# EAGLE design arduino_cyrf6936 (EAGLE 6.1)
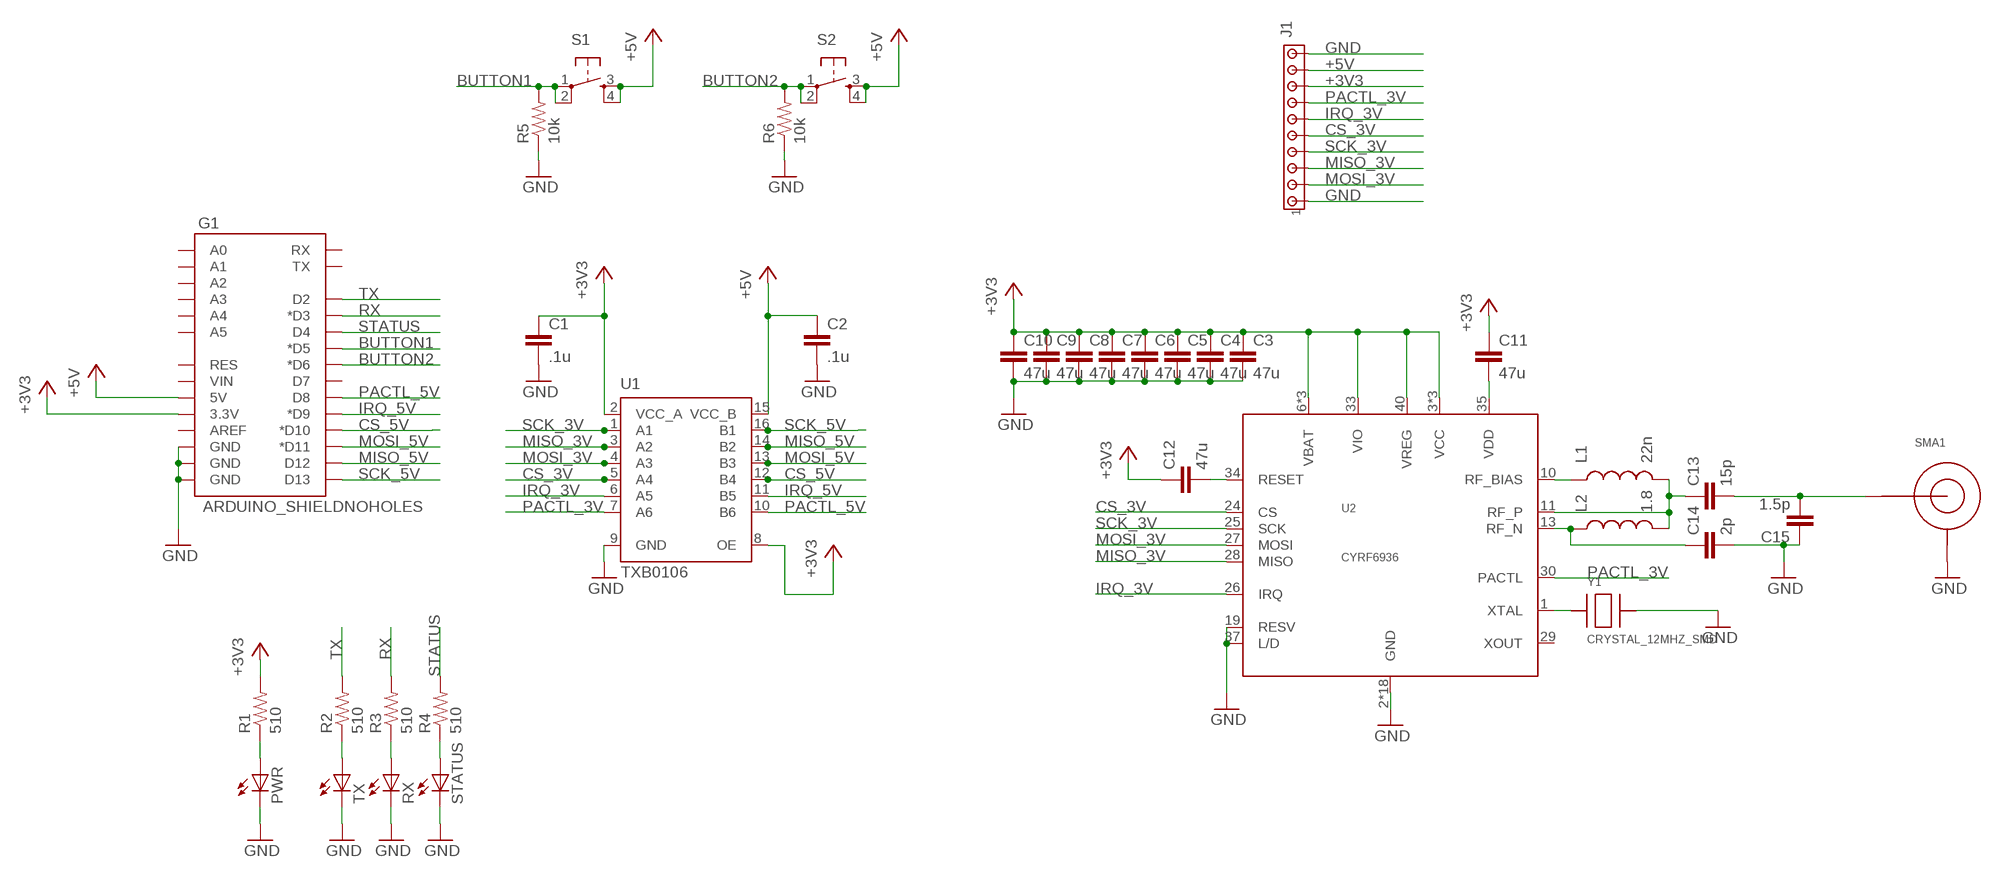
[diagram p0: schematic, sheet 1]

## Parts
C1  .1u  CAP0603-CAP  [0603-CAP]
C2  .1u  CAP0603-CAP  [0603-CAP]
C3  47u  CAP0603-CAP  [0603-CAP]
C4  47u  CAP0603-CAP  [0603-CAP]
C5  47u  CAP0603-CAP  [0603-CAP]
C6  47u  CAP0603-CAP  [0603-CAP]
C7  47u  CAP0603-CAP  [0603-CAP]
C8  47u  CAP0603-CAP  [0603-CAP]
C9  47u  CAP0603-CAP  [0603-CAP]
C10  47u  CAP0603-CAP  [0603-CAP]
C11  47u  CAP0603-CAP  [0603-CAP]
C12  47u  CAP0603-CAP  [0603-CAP]
C13  15p  CAP0402-CAP  [0402-CAP]
C14  2p  CAP0402-CAP  [0402-CAP]
C15  1.5p  CAP0402-CAP  [0402-CAP]
G1  ARDUINO_SHIELDNOHOLES  [DUEMILANOVE_SHIELD_NOHOLES]
J1  MTA10-100  [10X10MTA]
L1  22n  INDUCTOR0603  [0603]
L2  1.8  INDUCTOR0402  [C0402]
PWR  LED0603  [LED-0603]
R1  510  RESISTOR0603-RES  [0603-RES]
R2  510  RESISTOR0603-RES  [0603-RES]
R3  510  RESISTOR0603-RES  [0603-RES]
R4  510  RESISTOR0603-RES  [0603-RES]
R5  10k  RESISTOR0603-RES  [0603-RES]
R6  10k  RESISTOR0603-RES  [0603-RES]
RX  LED0603  [LED-0603]
S1  TAC_SWITCHSMD  [TACTILE_SWITCH_SMD]
S2  TAC_SWITCHSMD  [TACTILE_SWITCH_SMD]
SMA1  SMA_EDGE  [SMA_EDGE]
STATUS  LED0603  [LED-0603]
TX  LED0603  [LED-0603]
U1  TXB0106  [TSSOP16]
U2  CYRF6936  [QFN40-6X6]
Y1  CRYSTAL_12MHZ_SMD  [SMD-4_5X3.2MM]

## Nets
+3V3: C1.1 C3.1 C4.1 C5.1 C6.1 C7.1 C8.1 C9.1 C10.1 C11.1 C12.1 G1.3.3V J1.8 R1.2 U1.2(VCC_A) U1.8(OE) U2.3(VCC) U2.6(VBAT) U2.7(VCC) U2.8(VBAT) U2.16(VCC) U2.33(VIO) U2.38(VBAT) U2.40(VREG)
+5V: C2.1 G1.5V J1.9 S1.3 S1.4 S2.3 S2.4 U1.15(VCC_B)
BUTTON1: G1.D5(*D5) R5.2 S1.1 S1.2
BUTTON2: G1.D6(*D6) R6.2 S2.1 S2.2
CS_3V: J1.5 U1.5(A4) U2.24(CS)
CS_5V: G1.D10(*D10) U1.12(B4)
GND: C1.2 C2.2 C3.2 C4.2 C5.2 C6.2 C7.2 C8.2 C9.2 C10.2 C14.2 C15.1 G1.GND@0(GND) G1.GND@1(GND) G1.GND@2(GND) J1.1 J1.10 PWR.C R5.1 R6.1 RX.C SMA1.GND1(SHIELD) SMA1.GND2(SHIELD) STATUS.C TX.C U1.9(GND) U2.2(GND) U2.4(GND) U2.5(GND) U2.9(GND) U2.12(GND) U2.14(GND) U2.15(GND) U2.17(GND) U2.18(GND) U2.19(RESV) U2.20(GND) U2.21(GND) U2.22(GND) U2.23(GND) U2.31(GND) U2.32(GND) U2.36(GND) U2.37(L/D) U2.39(GND) U2.EXP(GND) Y1.P$3
IRQ_3V: J1.6 U1.6(A5) U2.26(IRQ)
IRQ_5V: G1.D9(*D9) U1.11(B5)
MISO_3V: J1.3 U1.3(A2) U2.28(MISO)
MISO_5V: G1.D12 U1.14(B2)
MOSI_3V: J1.2 U1.4(A3) U2.27(MOSI)
MOSI_5V: G1.D11(*D11) U1.13(B3)
N$1: PWR.A R1.1
N$2: R2.1 TX.A
N$3: R3.1 RX.A
N$4: R4.1 STATUS.A
N$5: L1.1 U2.10(RF_BIAS)
N$6: C13.1 L1.2 L2.2 U2.11(RF_P)
N$7: C11.2 U2.35(VDD)
N$8: C12.2 U2.34(RESET)
N$9: C14.1 L2.1 U2.13(RF_N)
N$10: U2.1(XTAL) Y1.P$1
N$11: C13.2 C15.2 SMA1.SIGNAL(CENTER)
PACTL_3V: J1.7 U1.7(A6) U2.30(PACTL)
PACTL_5V: G1.D8 U1.10(B6)
RX: G1.D3(*D3) R3.2
SCK_3V: J1.4 U1.1(A1) U2.25(SCK)
SCK_5V: G1.D13 U1.16(B1)
STATUS: G1.D4 R4.2
TX: G1.D2 R2.2
Unconnected: G1.A0 G1.A1 G1.A2 G1.A3 G1.A4 G1.A5 G1.AREF G1.D7 G1.RES G1.RX G1.TX G1.VIN U2.29(XOUT)

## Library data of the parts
C1-C15 = SparkFun-Passives:CAP: Capacitor
G1 = SparkFun-Boards:ARDUINO_SHIELD: Arduino shield footprint
J1 = con-amp:MTA10-100: AMP connector
L1 L2 = SparkFun-Passives:INDUCTOR: Inductors
PWR RX STATUS TX = SparkFun-LED:LED: LEDs
R1-R6 = SparkFun-Passives:RESISTOR: Resistor
S1 S2 = SparkFun-Electromechanical:TAC_SWITCH: Momentary Switch Button commonly used for reset or general input. Spark Fun Electronics SKU : COM-00097
SMA1 = DSS:SMA_EDGE: SMA edge connector, DigiKey part: J658-ND
U1 = DSS:TXB0106
U2 = DSS:CYRF6936: Cypress CYRF6936 2.4GHz DSSS radio. All N/C pins and the exposed pad are tied to ground.
Y1 = DSS:CRYSTAL_12MHZ_SMD: 12MHz crystal, SMD

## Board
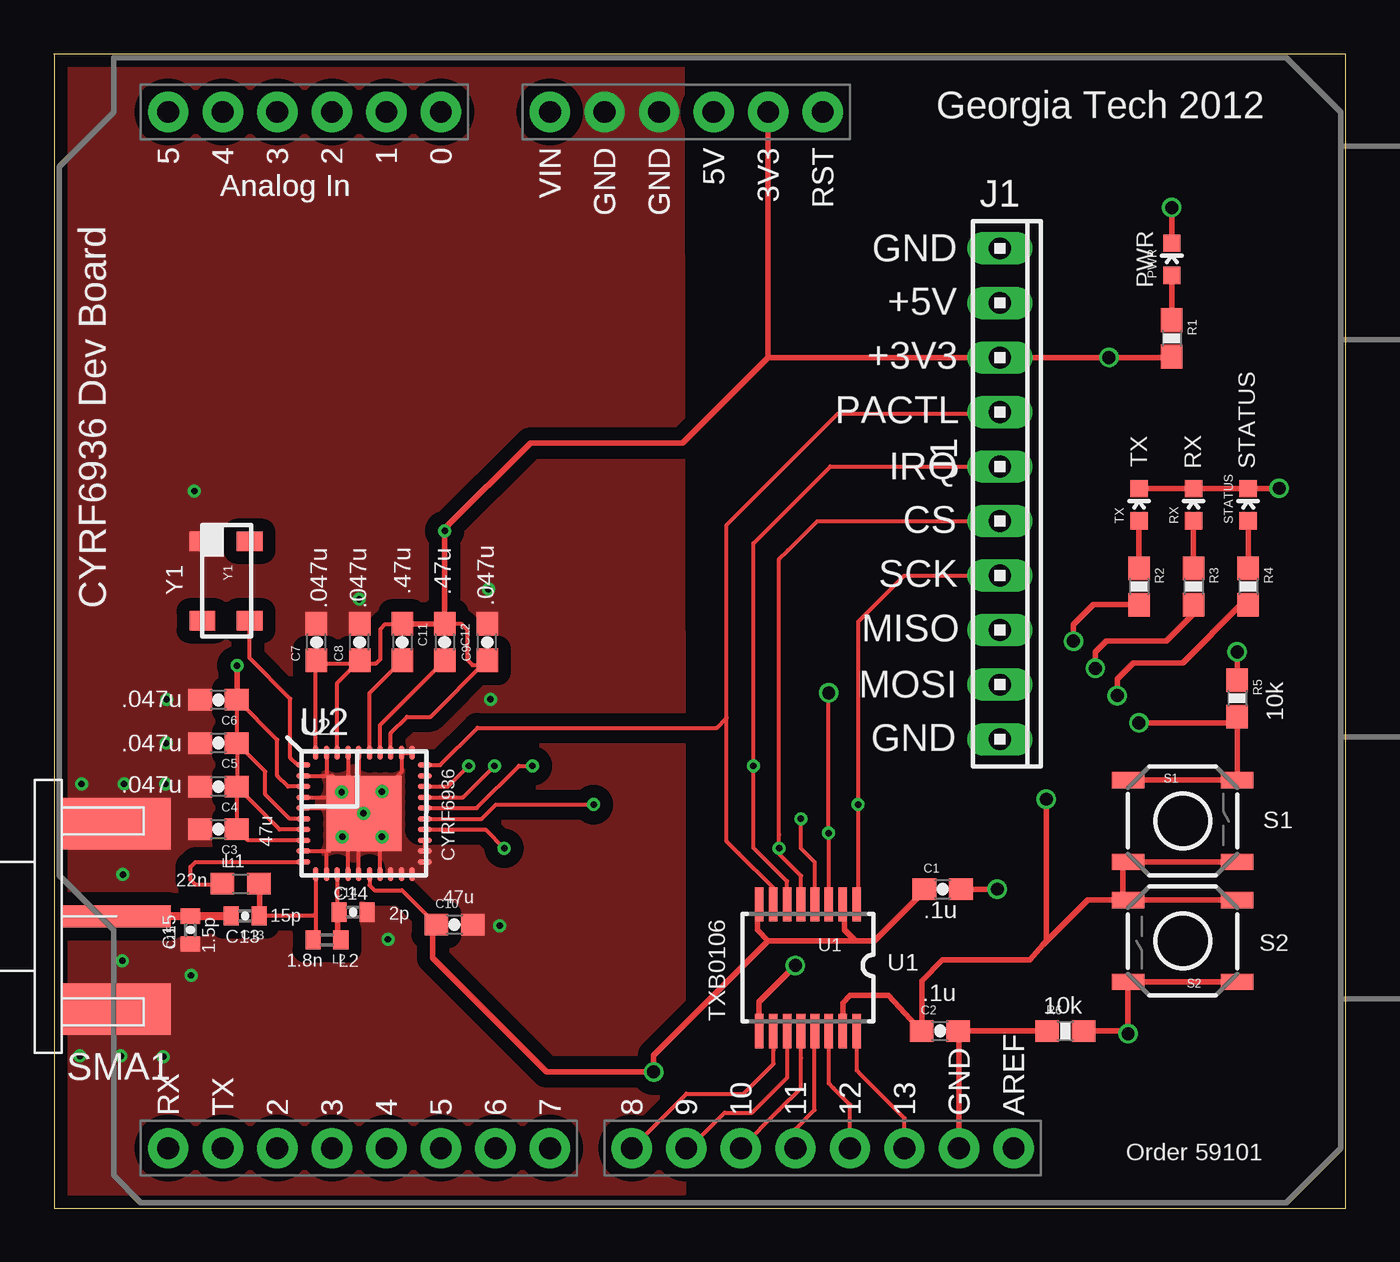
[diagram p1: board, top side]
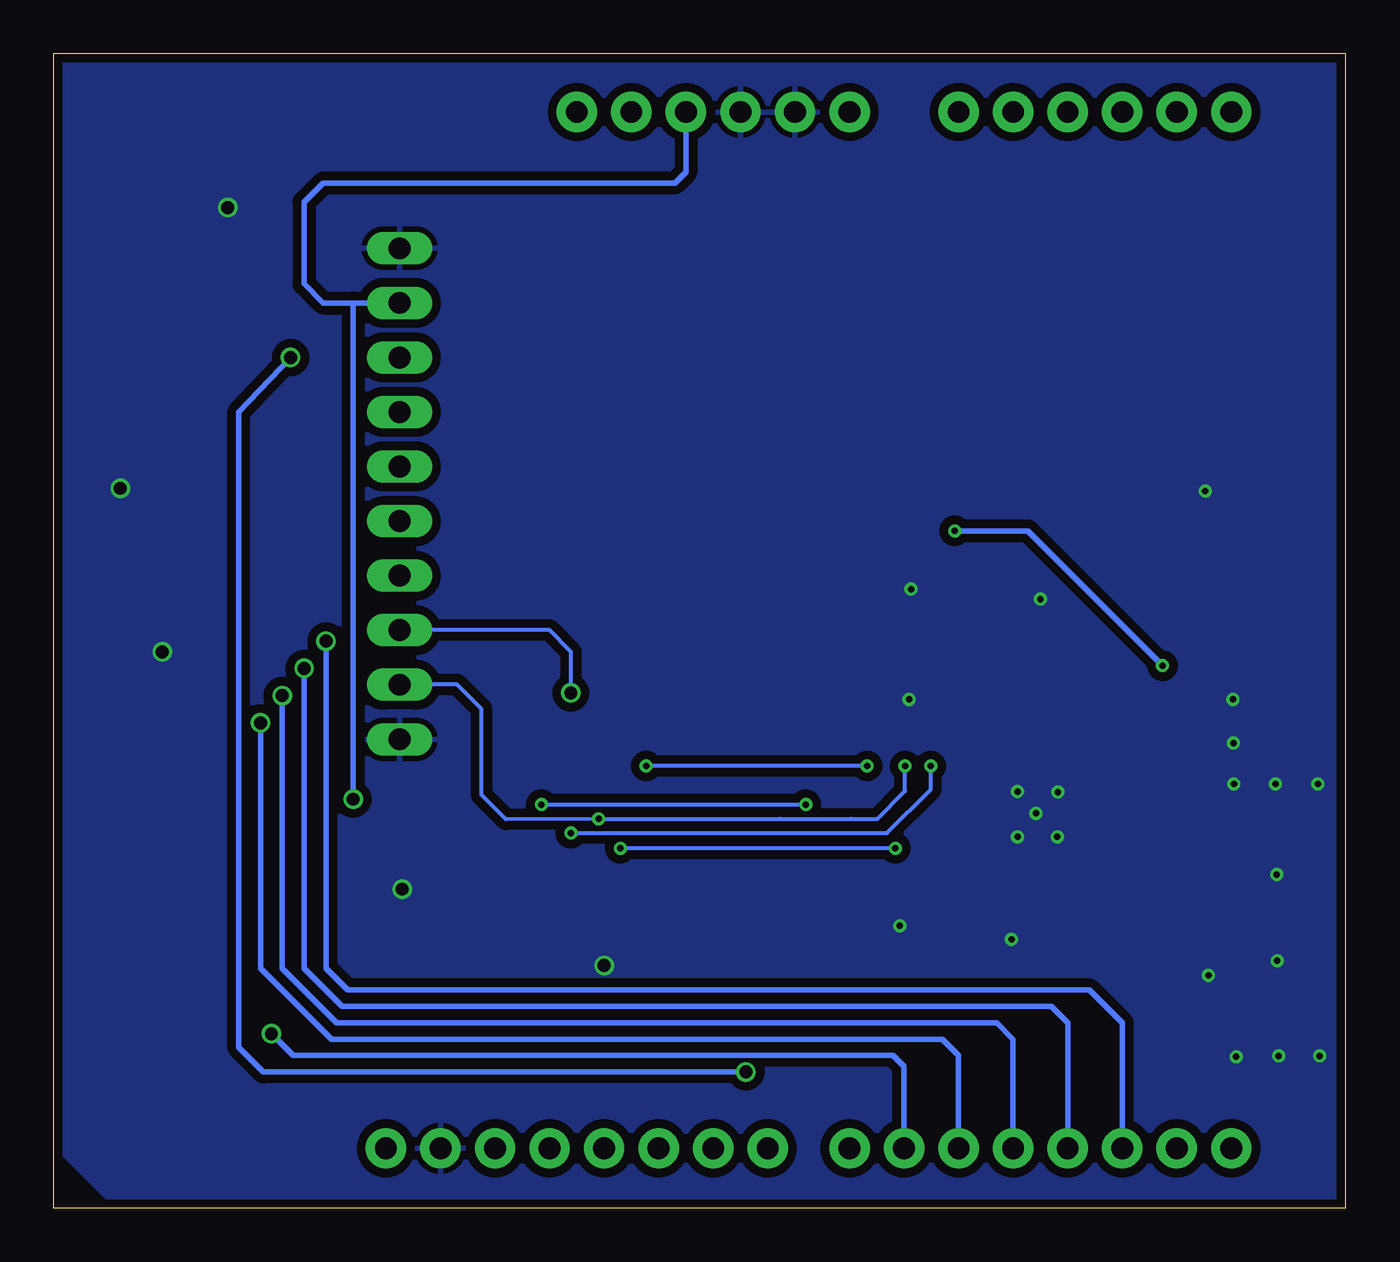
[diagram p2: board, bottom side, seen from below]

Size 60.18 x 53.77 mm. Coordinates in mm from the lower left corner, seen from the top.
Outline: 60.18,53.77 60.18,0 0.02,0 0.02,53.77
Outline: 60.18,53.77 60.18,53.77
Outline: 0,53.77 0.02,53.77
Outline: 0.02,53.77 60.18,53.77
Copper layers (1*16): Top 0.035mm / dielectric 1.5mm / Bottom 0.035mm
Design rules: minimum track width 6mil, minimum drill 12mil, track to track 6mil, track to pad 6mil, pad to pad 6mil, via to via 6mil, smd to smd 0mil, copper to edge 10mil, drill to drill 10mil, minimum pad ring 10mil, minimum via ring 6mil, stop-mask expansion 2mil, vias tented up to drill 100mil, thermal gap 10mil

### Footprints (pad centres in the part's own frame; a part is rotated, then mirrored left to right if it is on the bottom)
0603-CAP = smd 1.1 x 1: 1 -0.85,0; 2 0.85,0
0402-CAP = smd 0.7 x 0.9: 1 -0.65,0; 2 0.65,0
DUEMILANOVE_SHIELD_NOHOLES = drill 1.016 pad 1.88: 3.3V 50.8,26.67; 5V 50.8,29.21; A0 50.8,41.91; A1 50.8,44.45; A2 50.8,46.99; A3 50.8,49.53; A4 50.8,52.07; A5 50.8,54.61; AREF 2.54,15.24; D2 2.54,49.53; D3 2.54,46.99; D4 2.54,44.45; D5 2.54,41.91; D6 2.54,39.37; D7 2.54,36.83; D8 2.54,33.02; D9 2.54,30.48; D10 2.54,27.94; D11 2.54,25.4; D12 2.54,22.86; D13 2.54,20.32; GND@0 50.8,31.75; GND@1 50.8,34.29; GND@2 2.54,17.78; RES 50.8,24.13; RX 2.54,54.61; TX 2.54,52.07; VIN 50.8,36.83
10X10MTA = drill 1.016 long: 1 11.43,0; 2 8.89,0; 3 6.35,0; 4 3.81,0; 5 1.27,0; 6 -1.27,0; 7 -3.81,0; 8 -6.35,0; 9 -8.89,0; 10 -11.43,0
0603 = smd 1.1 x 1: 1 -0.85,0; 2 0.85,0
C0402 = smd 0.7 x 0.9: 1 -0.65,0; 2 0.65,0
LED-0603 = smd 0.8 x 0.8: A 0,-0.75; C 0,0.75
0603-RES = smd 1.1 x 1: 1 -0.85,0; 2 0.85,0
TACTILE_SWITCH_SMD = smd 1.524 x 0.762: 1 -2.54,1.905; 2 2.54,1.905; 3 -2.54,-1.905; 4 2.54,-1.905
SMA_EDGE = smd 2.413 x 5.08: GND1 -4.318,0; GND2 4.318,0 | smd 1.016 x 5.08: SIGNAL 0,0
TSSOP16 = smd 0.4 x 1.6: 1 -2.225,-2.85; 2 -1.575,-2.85; 3 -0.925,-2.85; 4 -0.275,-2.85; 5 0.375,-2.85; 6 1.025,-2.85; 7 1.675,-2.85; 8 2.325,-2.85; 9 2.325,3.05; 10 1.675,3.05; 11 1.025,3.05; 12 0.375,3.05; 13 -0.275,3.05; 14 -0.925,3.05; 15 -1.575,3.05; 16 -2.225,3.05
QFN40-6X6 = smd 0.65 x 0.25: 1 -2.825,2.25; 2 -2.825,1.75; 3 -2.825,1.25; 4 -2.825,0.75; 5 -2.825,0.25; 6 -2.825,-0.25; 7 -2.825,-0.75; 8 -2.825,-1.25; 9 -2.825,-1.75; 10 -2.825,-2.25; 21 2.825,-2.25; 22 2.825,-1.75; 23 2.825,-1.25; 24 2.825,-0.75; 25 2.825,-0.25; 26 2.825,0.25; 27 2.825,0.75; 28 2.825,1.25; 29 2.825,1.75; 30 2.825,2.25 | smd 0.25 x 0.65: 11 -2.25,-2.825; 12 -1.75,-2.825; 13 -1.25,-2.825; 14 -0.75,-2.825; 15 -0.25,-2.825; 16 0.25,-2.825; 17 0.75,-2.825; 18 1.25,-2.825; 19 1.75,-2.825; 20 2.25,-2.825; 31 2.25,2.825; 32 1.75,2.825; 33 1.25,2.825; 34 0.75,2.825; 35 0.25,2.825; 36 -0.25,2.825; 37 -0.75,2.825; 38 -1.25,2.825; 39 -1.75,2.825; 40 -2.25,2.825 | smd 3.5 x 3.5: EXP 0,0
SMD-4_5X3.2MM = smd 0.9 x 1.2: P$1 1.9,1.1; P$2 1.9,-1.1; P$3 -1.8,-1.1; P$4 -1.8,1.1

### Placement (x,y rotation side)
C1  41.4,14.86 0 top
C2  41.28,8.25 0 top
C3  7.67,17.65 180 top
C4  7.67,19.63 180 top
C5  7.67,21.67 180 top
C6  7.67,23.67 180 top
C7  12.24,26.37 90 top
C8  14.25,26.37 90 top
C9  20.19,26.37 90 top
C10  18.67,13.21 0 top
C11  16.23,26.37 270 top
C12  18.21,26.37 270 top
C13  8.92,13.61 180 top
C14  13.94,13.79 0 top
C15  6.38,12.95 90 top
G1  59.94,0.25 90 top
J1  44.07,33.27 270 top
L1  8.71,15.11 0 top
L2  12.73,12.5 180 top
PWR  52.07,44.2 0 top
R1  52.07,40.51 270 top
R2  50.55,28.96 270 top
R3  53.09,28.96 270 top
R4  55.63,28.96 270 top
R5  55.12,23.75 270 top
R6  47.12,8.25 0 top
RX  53.09,32.77 0 top
S1  52.58,18.03 0 top
S2  52.58,12.45 180 top
SMA1  2.92,13.59 90 top
STATUS  55.63,32.77 0 top
TX  50.55,32.77 0 top
U1  35.18,11.3 180 top
U2  14.45,18.39 0 top
Y1  8.03,29.26 270 top

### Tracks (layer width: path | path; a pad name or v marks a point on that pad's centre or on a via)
+3V3  (via drill 0.3, 0.6)
  Top 0.178: U2.8 9.03,17.14 C3.1 | U2.7 10.52,17.64 C4.1 8.53,19.65 8.53,19.84 | U2.6 10.99,18.14 9.86,19.28 9.86,20.33 C5.1 | C6.1 C5.1 | C5.1 8.52,21.6 8.53,21.59 8.53,19.84 | 8.53,17.58 8.53,17.63 8.53,19.84 | U2.3 10.92,19.64 10.41,20.14 10.41,21.82 8.53,23.7 | U2.40 12.2,25.47 C7.1 12.17,25.44 12.17,25.38 14.2,25.38 | U2.38 13.2,24.47 C8.1 14.2,25.46 14.2,25.38 | 20.17,25.5 17.55,22.88 16.46,22.88 15.7,22.13 U2.33 15.72,21.21 15.75,21.18 | U2.16 14.7,15.04 14.93,14.81 16.22,14.81 C10.1 | 14.2,25.38 15.01,25.38 15.21,25.58 15.21,26.97 15.44,27.2 16.22,27.2 C11.1 | 20.17,25.3 20.14,25.32 20.14,25.35 | C12.1 19,27.2 19.25,26.95 19.25,25.55 19.51,25.3 20.09,25.3 20.14,25.35 | 20.14,25.35 20.14,25.45 20.17,25.48 | 20.14,25.35 20.14,25.46 C9.1 | v27.94,6.35 27.91,6.35 | R1.2 52.07,39.62
  Top 0.254: G1.3.3V 33.27,39.62 | 33.27,39.62 29.29,35.64 22.2,35.64 18.21,31.65 v18.21,31.55 | 33.27,39.62 38.28,39.62 40.01,39.62 J1.8 v49.15,39.62 52.07,39.62 | 40.54,14.87 C1.1 40.55,14.77 38.23,12.45 37.47,12.45 | 37.47,12.45 37.34,12.45 36.83,12.95 36.83,13.97 36.7,14.1 | 36.7,14.1 36.83,14.22 | 36.7,14.1 U1.2 | 37.47,12.45 33.27,12.45 | 33.27,12.45 32.77,12.95 32.77,14.1 32.89,14.22 32.89,14.19 U1.8 | v27.94,6.35 27.94,7.11 33.27,12.45 | v18.21,31.55 C12.1 C11.1 | v8.53,25.27 8.53,23.7 8.53,23.69 C6.1 | v18.21,31.55 18.24,31.57 | C3.1 8.52,17.64 8.53,17.63 8.48,17.63 8.46,17.6 | 8.53,17.58 8.56,17.58 | C9.1 20.18,25.52 20.17,25.5 | 27.91,6.35 22.96,6.35 17.65,11.66 17.65,12.9 17.82,13.07 C10.1
  Bottom 0.254: v27.94,6.35 28.32,6.35 50.42,6.35 51.56,7.49 51.56,37.08 v49.15,39.62 | v8.53,25.27 14.81,31.55 v18.21,31.55
+5V  (via drill 0.6)
  Top 0.254: S1.4 S1.3 49.91,16.13 49.78,16 49.78,14.61 S2.4 | S2.4 S2.3 | 46.08,12.27 45.47,11.56 41.4,11.56 40.43,10.58 C2.1 40.41,8.24 38.88,9.91 37.08,9.91 36.75,9.58 U1.15 | 46.08,12.27 46.23,12.45 v46.23,19.05 | S2.4 48.16,14.35 46.08,12.27
  Bottom 0.178: J1.9 44.04,42.16
  Bottom 0.254: G1.5V 30.73,48.26 31.24,47.75 47.62,47.75 48.51,46.86 48.51,43.05 47.62,42.16 46.23,42.16 | 46.23,42.16 J1.9 44.04,42.16 43.94,42.16 | 46.23,42.16 v46.23,19.05
BUTTON1  (via drill 0.6)
  Top 0.254: S1.1 S1.2 55.12,22.61 | v50.55,22.61 55.12,22.61 | 55.12,22.61 55.12,22.86 R5.2 55.12,22.99
  Bottom 0.254: G1.D5 18.03,7.11 18.8,7.87 47.24,7.87 50.55,11.18 v50.55,22.61
BUTTON2  (via drill 0.6)
  Top 0.254: 50.04,10.41 v50.04,8.13 49.91,8.25 R6.2 | S2.1 S2.2 | S2.2 49.91,10.54 50.04,10.41 | S2.2 50.04,10.41
  Bottom 0.254: G1.D6 20.57,6.6 21.08,7.11 49.02,7.11 v50.04,8.13
CS_3V  (via drill 0.3)
  Top 0.178: U1.5 34.8,15.49 33.83,16.46 33.78,16.51 v33.78,16.76 33.78,17.4 33.78,30.23 34.19,30.63 35.56,32 J1.5 | U2.24 20.11,17.64 v20.98,16.76
  Bottom 0.178: v20.98,16.76 v33.78,16.76
CS_5V
  Top 0.178: G1.D10 33.78,4.57 34.8,5.59 34.8,6.99 U1.12
GND  (via drill 0.3, 0.6)
  Top 0.178: U2.9 12.83,16.64 13.46,17.27 | U2.12 12.7,16.56 v13.44,17.3 13.7,17.03 U2.14 | U2.17 15.2,16.81 | 15.2,16.81 15.2,17.21 v15.29,17.3 | U2.15 14.2,16.72 14.27,16.79 14.27,16.71 15.1,16.71 15.2,16.81 | U2.4 13.17,19.14 v13.41,19.38 | U2.5 12.93,18.64 13.11,18.47 | U2.2 12.75,20.14 | 12.75,20.14 12.98,20.14 13.23,19.89 13.23,19.56 v13.41,19.38 | U2.39 12.7,20.19 12.75,20.14 | U2.37 13.7,20.18 13.84,20.04 13.84,19.79 13.46,19.41 | U2.36 14.2,20.17 v13.41,19.38 | U2.32 16.2,20.32 v15.29,19.41 | 16.23,21.21 U2.31 | U2.23 U2.22
  Top 0.254: 52.32,44.96 52.07,44.96 PWR.C v52.07,46.61 | TX.C RX.C STATUS.C v57.07,33.53 | G1.GND@2 42.16,8.25 | 42.16,8.25 46.1,8.25 | 46.1,8.25 R6.1 | R6.1 46.48,8.25 | C1.2 v43.94,14.86 | R5.1 v55.12,25.91 | C2.2 42.16,8.25 | R6.1 46.1,8.25 | U1.9 32.85,9.61 v34.54,11.3
  other vias: 6.55,33.4 5.26,23.7 14.22,28.37 20.78,13.16 6.4,10.85 3.28,19.76 15.57,12.52 5.11,7.06 20.24,28.83 5.23,21.67 5.21,19.76 14.43,18.39 1.3,19.76 1.22,7.09 20.35,23.7 3.12,7.09 3.23,15.54 3.2,11.53
  pour Bottom (isolate 0.406): 0.51,53.59 0.51,0.25 57.4,0.25 59.94,2.79 60.02,53.7
  pour Top (isolate 0.61, no thermals): 0.51,53.21 0.51,0.51 29.34,0.69 29.26,53.16
IRQ_3V  (via drill 0.3)
  Top 0.178: U2.26 19.53,18.64 19.71,18.64 21.67,20.6 v22.3,20.6 | U1.6 34.15,15.22 33.53,15.85 32.59,16.79 v32.59,20.6 32.59,30.96 36.17,34.54 J1.6
  Bottom 0.178: v22.3,20.6 v32.59,20.6
IRQ_5V
  Top 0.178: U1.11 34.16,7.24 34.16,6.1 32.51,4.44 31.24,4.44 29.59,2.79 G1.D9
  Top 0.254: U1.11
MISO_3V  (via drill 0.3, 0.6)
  Top 0.178: U1.3 36.1,17.36 v36.09,17.47 v36.09,24 | U2.28 18.36,19.63 v19.33,20.6
  Top 0.254: U2.28
  Bottom 0.178: v36.09,17.47 27.56,17.47 21.36,17.47 19.33,19.51 v19.33,20.6 | v36.09,24 36.09,25.91 37.08,26.92 J1.3
  Bottom 0.254: J1.3 44.2,26.92 J1.3
MISO_5V
  Top 0.178: G1.D12 37.08,4.83 36.32,5.59 36.1,5.81 U1.14
MOSI_3V  (via drill 0.3)
  Top 0.178: U1.4 35.45,16.11 34.8,16.76 v34.8,18.14 | U2.27 19.06,19.14 v20.52,20.6
  Bottom 0.178: J1.2 41.4,24.38 40.26,23.24 40.26,19.25 39.12,18.11 v34.8,18.14 26.36,18.14 23.04,18.14 21.82,18.14 20.52,19.43 v20.52,20.6
MOSI_5V
  Top 0.178: G1.D11 34.54,3.68 35.43,4.57 35.43,8.13 | U1.13 35.45,8.28 35.46,8.28 35.43,8.25
  Top 0.254: 35.43,8.13 35.43,8.25
N$1
  Top 0.254: PWR.A R1.1
N$2
  Top 0.254: TX.A R2.1
N$3
  Top 0.254: RX.A R3.1
N$4
  Top 0.254: STATUS.A R4.1
N$5
  Top 0.178: 7.74,15.06 6.6,15.06 6.37,15.29 6.37,15.9 6.6,16.13 11.61,16.13
  Top 0.254: L1.1 7.74,15.06 | U2.10 11.63,16.13 11.66,16.13 11.61,16.13
N$6
  Top 0.178: U2.11 12.2,13.56 | 12.2,13.56 12.2,12.63 | 12.2,12.63 12.19,12.62 | 12.19,12.62 L2.2 | 9.6,13.65 12.12,13.65 12.2,13.56 | 12.19,12.62 12.2,12.63
  Top 0.254: 12.19,12.68 12.19,12.62 | L2.2 12.09,12.5 12.09,12.55 12.17,12.55 12.19,12.62 | 12.19,12.62 12.17,12.68 12.17,12.72 12.17,12.7 12.19,12.68 | C13.1 9.6,13.65 9.6,15.14 9.56,15.18 L1.2 | 12.19,12.62 12.19,12.68
N$7
  Top 0.178: U2.35 14.7,23.99 C11.2
N$8
  Top 0.178: U2.34 15.2,22.51 C12.2
N$9
  Top 0.178: U2.13 13.19,13.79
  Top 0.254: 13.19,13.79 C14.1 13.23,13.79 | L2.1 13.23,12.45 13.23,13.79 | 13.23,13.79 13.23,13.84 | 13.23,13.84 13.23,13.79 | 13.23,13.79 13.23,13.84
N$10
  Top 0.178: U2.1 11.36,20.64 11.02,20.98 11.02,23.72 9.12,25.63 9.12,27.33 9.12,27.35 Y1.P$1
N$11
  Top 0.254: C13.2 7.54,13.6 C15.2
  Top 0.406: C13.2 SMA1.SIGNAL
PACTL_3V
  Top 0.178: U2.30 18,20.64 19.74,22.38 30.89,22.38 31.34,22.83 | U1.7 33.5,14.93 31.9,16.54 31.34,17.09 31.34,22.83 | 31.34,22.83 31.34,31.83 36.53,37.01 43.99,37.01 J1.7
PACTL_5V
  Top 0.178: G1.D8 29.46,5.33 32.13,5.33 33.53,6.73 33.53,7.37 33.53,8.15
  Top 0.254: 33.53,8.15 U1.10
RX  (via drill 0.6)
  Top 0.254: R3.2 53.09,27.69 51.82,26.42 49.02,26.42 48.51,25.91 v48.51,25.15
  Bottom 0.254: G1.D3 12.95,8.64 13.72,9.4 46.74,9.4 48.51,11.18 v48.51,25.15
SCK_3V  (via drill 0.3)
  Top 0.178: 37.47,14.34 v37.47,18.8 37.47,27.3 39.62,29.46 J1.4 | U2.25 19.94,18.14 20.6,18.8 25.09,18.8
  Top 0.254: 37.47,14.34 U1.1 | U2.25 | 25.09,18.8 25.12,18.8 v25.15,18.8
  Bottom 0.178: v37.47,18.8 v25.15,18.8
SCK_5V
  Top 0.178: G1.D13 39.62,4.19 37.59,6.22 37.4,6.41 U1.16
STATUS  (via drill 0.6)
  Top 0.254: R4.2 55.28,28.11 52.58,25.4 50.29,25.4 49.53,24.64 v49.53,23.88
  Bottom 0.254: G1.D4 15.49,7.87 16.26,8.64 46.99,8.64 49.53,11.18 v49.53,23.88
TX  (via drill 0.6)
  Top 0.254: R2.2 48.43,28.11 47.5,27.18 v47.5,26.42
  Bottom 0.254: G1.D2 10.41,8.64 11.94,10.16 46.48,10.16 47.5,11.18 v47.5,26.42

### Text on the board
_tsilk: Georgia Tech 2012 | 5 | 4 | 3 | 2 | 1 | 0 | VIN | GND | GND | 5V | 3V3 | RST | Analog In | J1 | CYRF6936 Dev Board | GND | PWR | +5V | +3V3 | PACTL | TX | RX | STATUS | IRQ | CS | Y1 | .047u | .047u | .47u | .47u | .047u | SCK | MISO | .047u | 10k | MOSI | .047u | U2 | GND | .047u | S1 | 47u | CYRF6936 | 22n | L1 | 15p | C14 | 47u | C13 | 2p | TXB0106 | .1u | C15 | S2 | 1.5p | 1.8n | L2 | U1 | .1u | 10k | RX | TX | 2 | 3 | 4 | 5 | 6 | 7 | 8 | 9 | 10 | 11 | 12 | 13 | GND | AREF | Order 59101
